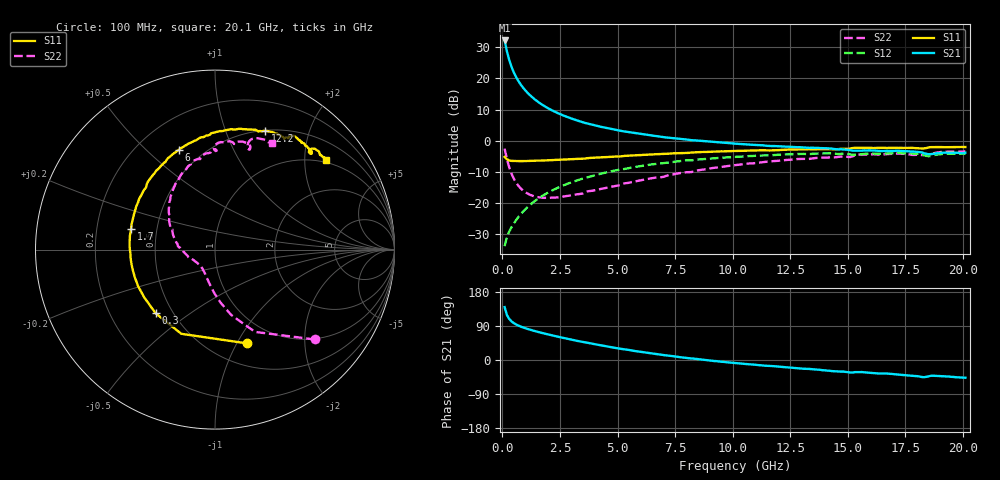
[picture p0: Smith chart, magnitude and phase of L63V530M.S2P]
!  Infineon Technologies AG
! BFR380L3 , PF131585-7, No.6, Th 09.10.01, soldered on pcb-board, measured with PP GSG850
!  Vce=3.5 V,  Ic=30.0 mA
! Common Emitter S-Parameters:  15. November 2001
#  GHz  S  MA  R  50
! f  S11  S21  S12  S22
! GHz  Mag  Ang  Mag  Ang  Mag  Ang  Mag  Ang
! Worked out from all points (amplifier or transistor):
!   201 points, 100 MHz to 20.1 GHz, reference 50 ohm
!   highest |S21| = 32.2 dB at 100 MHz (marker M1)
!   |S21| within 3 dB of that: start of sweep to 186.8 MHz
!   unconditionally stable (mu >= 1): 1.207 GHz to 4.355 GHz
!   at 3.4 GHz: K = 1.02, MAG = 8.4 dB, |S12| = -12.3 dB
!   at 10.1 GHz: K = 0.96, MSG = 2.1 dB, |S12| = -5.2 dB
!   at 20.1 GHz: K = 0.98, MSG = 0.1 dB, |S12| = -4.1 dB
!   S11 on the Smith chart (normalised r, x): 100 MHz: 0.73, -1.10; 300 MHz: 0.40, -0.37; 1.7 GHz: 0.35, +0.10; 6 GHz: 0.37, +0.63; 12.2 GHz: 0.51, +1.38; 20.1 GHz: 0.93, +2.52
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0.1  0.5507 -71.4  40.54 139.4  0.02046 63.5  0.7483 -42.0
0.2  0.5053 -111.8  27.23 118.8  0.02867 56.4  0.5098 -64.1
0.3  0.4852 -132.9  19.74 108.4  0.0352 56.8  0.3748 -76.1
0.4  0.4758 -145.8  15.32 101.9  0.04114 58.1  0.2961 -84.1
0.5  0.4746 -154.7  12.46 97.2  0.04725 60.5  0.2469 -90.3
0.6  0.4726 -161.2  10.48 93.7  0.05355 62.2  0.2135 -95.3
0.7  0.4721 -166.5  9.059 90.8  0.06002 63.5  0.1897 -99.7
0.8  0.4723 -170.6  7.958 88.2  0.0667 64.6  0.1725 -103.6
1  0.4719 -177.3  6.419 83.8  0.08008 65.9  0.1497 -110.6
1.2  0.4764 177.3  5.381 80.0  0.09375 66.4  0.1364 -116.7
1.4  0.4787 172.5  4.635 76.5  0.1075 66.4  0.1283 -122.2
1.7  0.4813 166.5  3.849 71.7  0.1282 65.8  0.1229 -129.7
2.4  0.4943 154.3  2.785 61.6  0.1761 62.8  0.1239 -144.1
3.5  0.5171 138.1  1.978 47.5  0.2489 56.2  0.1435 -160.7
4.8  0.5556 122.7  1.529 33.0  0.3279 47.6  0.1855 179.8
6  0.5902 110.1  1.287 21.5  0.3929 39.3  0.2325 165.2
6.8  0.6115 102.5  1.171 14.4  0.4328 33.5  0.2606 155.7
10.1  0.6874 78.2  0.9007 -8.0  0.5519 12.0  0.407 125.2
12.2  0.7172 67.2  0.8077 -18.6  0.6021 -0.7  0.4875 107.9
13.5  0.7314 60.9  0.7733 -24.6  0.6189 -8.5  0.5226 98.6
16.8  0.7703 48.5  0.6901 -36.4  0.6273 -24.5  0.6151 77.9
20.1  0.7941 39.0  0.6434 -46.8  0.622 -38.2  0.6738 61.8
